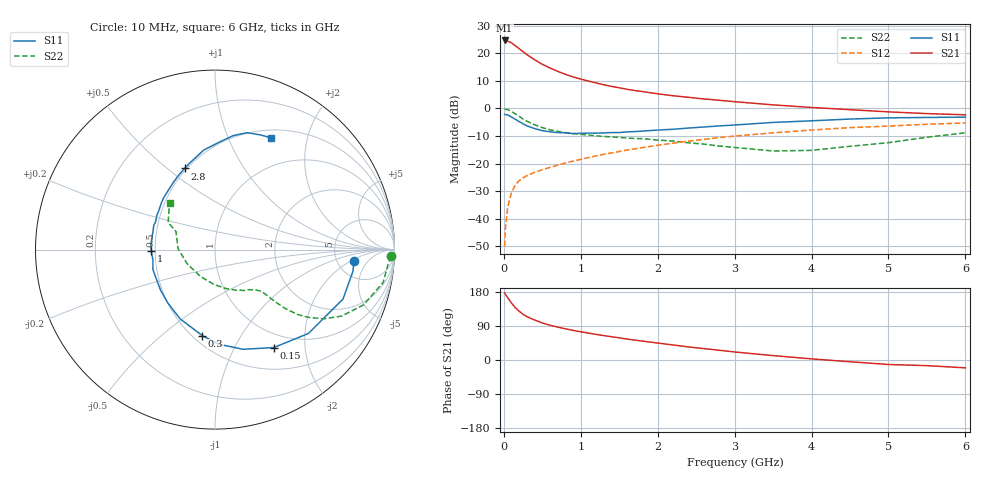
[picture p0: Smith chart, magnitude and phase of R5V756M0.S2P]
! SIEMENS Small Signal Semiconductors
! BFR183
! Si NPN RF Bipolar Junction Transistor in SOT23
! VCE = 0.75 V  IC = 6 mA
! Common Emitter S-Parameters:  May  1996
# GHz  S  MA  R  50
!  f  S11  S21  S12  S22
! GHz  MAG  ANG  MAG  ANG  MAG  ANG  MAG  ANG
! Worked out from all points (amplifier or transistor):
!   36 points, 10 MHz to 6 GHz, reference 50 ohm
!   highest |S21| = 24.6 dB at 10 MHz (marker M1)
!   |S21| within 3 dB of that: start of sweep to 201.1 MHz
!   unconditionally stable (mu >= 1): 871.1 MHz to 3.002 GHz
!   at 250 MHz: K = 0.48, MSG = 22.9 dB, |S12| = -25.2 dB
!   at 1.4 GHz: K = 1.08, MAG = 10.3 dB, |S12| = -16.1 dB
!   at 6 GHz: K = 0.95, MSG = 1.5 dB, |S12| = -5.3 dB
!   S11 on the Smith chart (normalised r, x): 10 MHz: 7.25, -2.28; 150 MHz: 0.79, -1.46; 300 MHz: 0.56, -0.70; 1 GHz: 0.48, -0.01; 2.8 GHz: 0.49, +0.58; 6 GHz: 0.60, +1.45
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0.01  0.7773 -4.6  17.08 177.1  0.0032 90.1  0.9817 -2.2
0.02  0.7778 -9.0  16.99 173.4  0.0066 88.0  0.9692 -4.4
0.05  0.7646 -21.1  16.59 164.4  0.0162 78.9  0.9547 -11.0
0.1  0.6995 -41.9  15.45 150.2  0.0302 70.6  0.8835 -20.4
0.15  0.6366 -59.0  13.65 137.9  0.0412 63.4  0.7966 -27.7
0.2  0.5772 -74.2  12.12 128.5  0.0494 59.4  0.7181 -32.5
0.25  0.5273 -87.9  10.69 120.5  0.0552 56.4  0.6442 -35.9
0.3  0.4847 -98.4  9.449 114.5  0.0607 54.5  0.5865 -38.1
0.4  0.4321 -116.7  7.638 105.5  0.0698 53.1  0.5067 -40.1
0.5  0.3968 -131.6  6.31 97.8  0.0776 53.1  0.4499 -40.8
0.6  0.3781 -143.4  5.404 91.8  0.0856 53.6  0.4114 -41.2
0.7  0.3655 -153.7  4.716 86.8  0.094 54.5  0.3855 -41.3
0.8  0.363 -162.4  4.159 82.3  0.1026 54.7  0.3649 -41.7
1  0.3553 -178.5  3.408 74.4  0.1198 55.6  0.3402 -42.5
1.1  0.3582 175.2  3.137 71.0  0.129 55.8  0.3296 -43.7
1.6  0.3761 149.5  2.228 55.3  0.1762 54.8  0.2914 -50.0
2.2  0.42 128.4  1.7 39.7  0.2358 50.7  0.2566 -62.3
2.8  0.4829 110.5  1.408 25.7  0.2967 44.7  0.2088 -81.6
3.5  0.5583 96.4  1.163 11.6  0.362 35.9  0.1698 -118.9
4.5  0.6433 80.9  0.951 -4.6  0.45 22.9  0.2062 178.3
5.5  0.6875 68.3  0.808 -14.9  0.5171 11.1  0.3012 150.0
6  0.6967 63.2  0.768 -20.7  0.5463 3.4  0.3623 134.4
